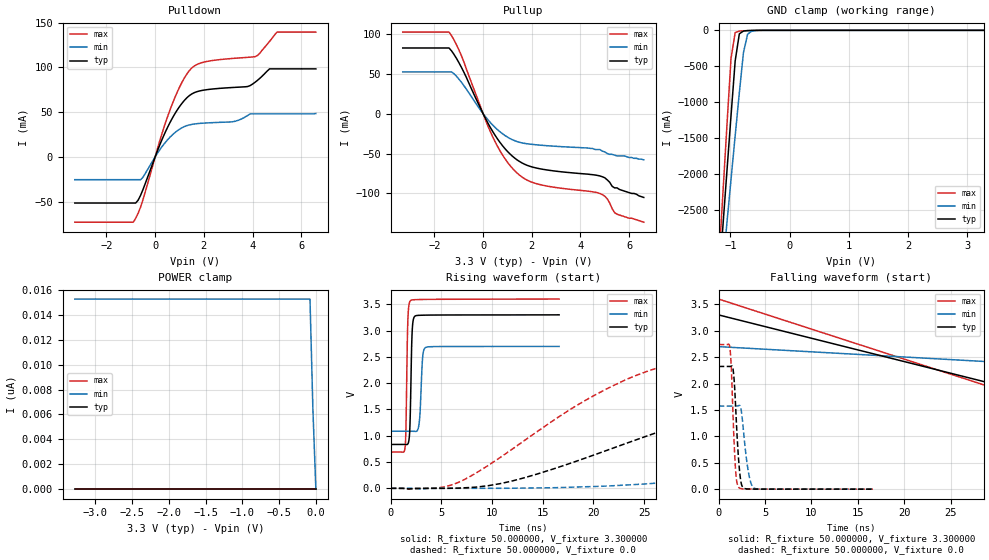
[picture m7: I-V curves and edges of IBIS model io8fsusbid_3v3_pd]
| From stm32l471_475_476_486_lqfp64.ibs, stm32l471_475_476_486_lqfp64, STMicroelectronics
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|   Model io8fsusbid_3v3_pd
[Model]  io8fsusbid_3v3_pd
Model_type I/O
Polarity   Non-Inverting
Enable   Active-Low
Vinl =   0.990000V
Vinh =   2.310000V
Vmeas =  1.650000V
Cref =   100.000000nF
Rref =   1.000000k
Vref =   3.300000V
C_comp   2.116400pF   2.092700pF   2.152900pF
[Temperature Range]   25.000000   0.125000k   -40.000000
[Pullup Reference]   3.300000V   2.700000V   3.600000V
[Pulldown Reference]   0.0V   0.0V   0.0V
[POWER Clamp Reference]   3.300000V   2.700000V   3.600000V
[GND Clamp Reference]   0.0V   0.0V   0.0V
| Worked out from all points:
|   slope of the pulldown table from 0 to 0.495 V, typ, clamps not added: 15.4 ohm
|   slope of the pullup table from 0 to 0.495 V, typ, clamps not added: 18.1 ohm
|   GND clamp passes 1 mA (typ) near -0.59 V on its own axis
|   rising waveform, R_fixture 50.000000, V_fixture 3.300000: 20-80 % time 165ps typ, 225ps min, 149ps max; typ from 0.835 V to 3.3 V
|   rising waveform, R_fixture 50.000000, V_fixture 0.0: 20-80 % time 23.9ns typ, 53.3ns min, 14.3ns max; typ from 0 V to 2.32 V
|   falling waveform, R_fixture 50.000000, V_fixture 3.300000: 20-80 % time 33.5ns typ, 61.1ns min, 30.7ns max; typ from 3.3 V to 0.835 V
|   falling waveform, R_fixture 50.000000, V_fixture 0.0: 20-80 % time 449ps typ, 626ps min, 371ps max; typ from 2.32 V to 0 V
[Pulldown]
|Voltage   I(typ)   I(min)   I(max)
-3.3V     -51.63mA   -25.53mA   -73.04mA
-900mV    -51.63mA   -25.53mA   -73.04mA
-500mV    -36.51mA   -22.8mA    -47.71mA
200mV     14.02mA    8.316mA    18.9mA
700mV     42.99mA    24.4mA     58.9mA
1.2V      63.06mA    33.8mA     88.14mA
1.6V      71.63mA    36.67mA    101.4mA
3.2V      77.51mA    39.29mA    110mA
4.1V      83.27mA    48mA       111.9mA
4.7V      98.3mA     48mA       129mA
5V        98.3mA     48mA       139.4mA
6.6V      98.3mA     48.43mA    139.4mA
[Pullup]
|Voltage   I(typ)   I(min)   I(max)
-3.3V     82.22mA    52.22mA    102.1mA
-1.4V     82.22mA    52.22mA    102.1mA
-900mV    58.55mA    39.64mA    73.33mA
100mV     -6.166mA   -3.962mA   -8.038mA
500mV     -27.53mA   -17.49mA   -35.6mA
1V        -47.29mA   -29.37mA   -60.81mA
1.5V      -60.05mA   -35.95mA   -77.15mA
2.4V      -69.45mA   -39.66mA   -89.34mA
4.8V      -78.1mA    -45mA      -100.1mA
5.1V      -83mA      -50mA      -106.7mA
5.5V      -93mA      -53mA      -126mA
6.6V      -105mA     -58mA      -136mA
[GND_clamp]
|Voltage   I(typ)   I(min)   I(max)
-3.3V     -9.914A    -9.595A    -9.188A
-1.2V     -3.541A    -3.911A    -3.279A
-1.13V    -2.75A     -3.295A    -2.301A
-1.06V    -1.963A    -2.68A     -1.33A
-990mV    -1.183A    -2.069A    -386.7mA
-920mV    -424.7mA   -1.463A    -31.42mA
-850mV    -49.13mA   -868.7mA   -10.49mA
-780mV    -9.132mA   -308.3mA   -6.726mA
-710mV    -3.661mA   -53.82mA   -3.996mA
-640mV    -1.738mA   -11.05mA   -1.896mA
-430mV    -33.31uA   -129.6uA   -18.85uA
3.28V     86.93uA    88.78uA    71.45uA
[POWER_clamp]
|Voltage   I(typ)   I(min)   I(max)
-3.28V    0A         15.27nA    0A
-80mV     0A         15.27nA    0A
-40mV     0A         6.354nA    0A
0V        0A         0A         0A
[Ramp]
| variable   typ   min   max
dV/dt_r  1.39404/23.91093n   0.94416/53.26977n   1.64262/14.30157n
dV/dt_f  1.47860/21.09034n   0.96750/44.71088n   1.74566/13.58933n
R_load = 50.000000
[Rising Waveform]
R_fixture= 50.000000
V_fixture= 3.300000
V_fixture_min= 2.700000
V_fixture_max= 3.600000
|time   V(typ)   V(min)   V(max)
0s        834.7mV    1.086V     689.8mV
1.401ns   834.1mV    1.086V     751.3mV
1.502ns   833.5mV    1.086V     1.116V
1.702ns   846.8mV    1.086V     3.237V
1.969ns   1.728V     1.086V     3.572V
2.135ns   3.042V     1.085V     3.583V
2.402ns   3.275V     1.082V     3.587V
2.803ns   3.29V      1.23V      3.59V
3.437ns   3.293V     2.677V     3.592V
16.62ns   3.299V     2.699V     3.599V
[Rising Waveform]
R_fixture= 50.000000
V_fixture= 0.0
V_fixture_min= 0.0
V_fixture_max= 0.0
|time   V(typ)   V(min)   V(max)
0s        3.142nV    58.62nV    2.998nV
6.607ns   3.524mV    -131.4uV   106.9mV
13.21ns   202.3mV    4.86mV     911.6mV
19.22ns   576.9mV    29.88mV    1.674V
25.23ns   991.2mV    84.9mV     2.22V
38.44ns   1.736V     312.3mV    2.613V
58.26ns   2.177V     728mV      2.711V
86.49ns   2.289V     1.197V     2.734V
112.9ns   2.314V     1.42V      2.737V
299.1ns   2.323V     1.574V     2.738V
[Falling Waveform]
R_fixture= 50.000000
V_fixture= 3.300000
V_fixture_min= 2.700000
V_fixture_max= 3.600000
|time   V(typ)   V(min)   V(max)
0s        3.299V     2.699V     3.599V
50.05ns   1.088V     2.207V     752.5mV
100.1ns   862.5mV    1.296V     694.5mV
150.2ns   839.9mV    1.146V     690.2mV
200.2ns   835.7mV    1.105V     689.8mV
300.3ns   834.7mV    1.089V     689.8mV
4.955us   834.7mV    1.086V     689.8mV
[Falling Waveform]
R_fixture= 50.000000
V_fixture= 0.0
V_fixture_min= 0.0
V_fixture_max= 0.0
|time   V(typ)   V(min)   V(max)
0s        2.323V     1.574V     2.738V
1.201ns   2.323V     1.574V     2.69V
1.368ns   2.329V     1.574V     2.3V
1.535ns   2.292V     1.574V     1.487V
1.802ns   1.675V     1.573V     440.2mV
2.202ns   452.5mV    1.586V     27.12mV
2.569ns   45.42mV    1.302V     5.93mV
3.203ns   3.672mV    331.3mV    2.159mV
3.804ns   1.6mV      20.25mV    1.327mV
16.62ns   3.142nV    58.62nV    2.998nV
